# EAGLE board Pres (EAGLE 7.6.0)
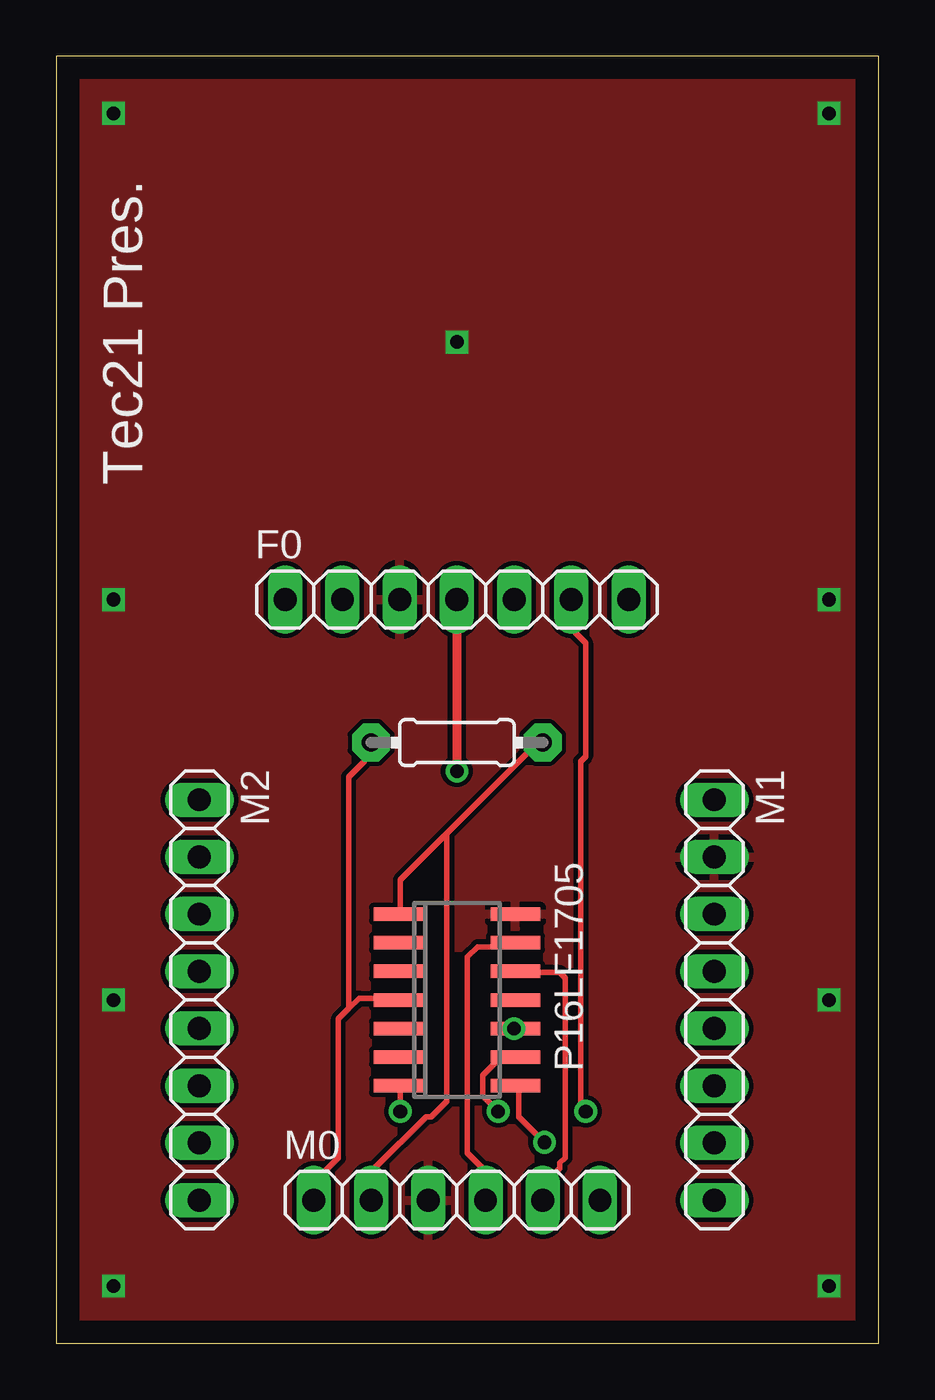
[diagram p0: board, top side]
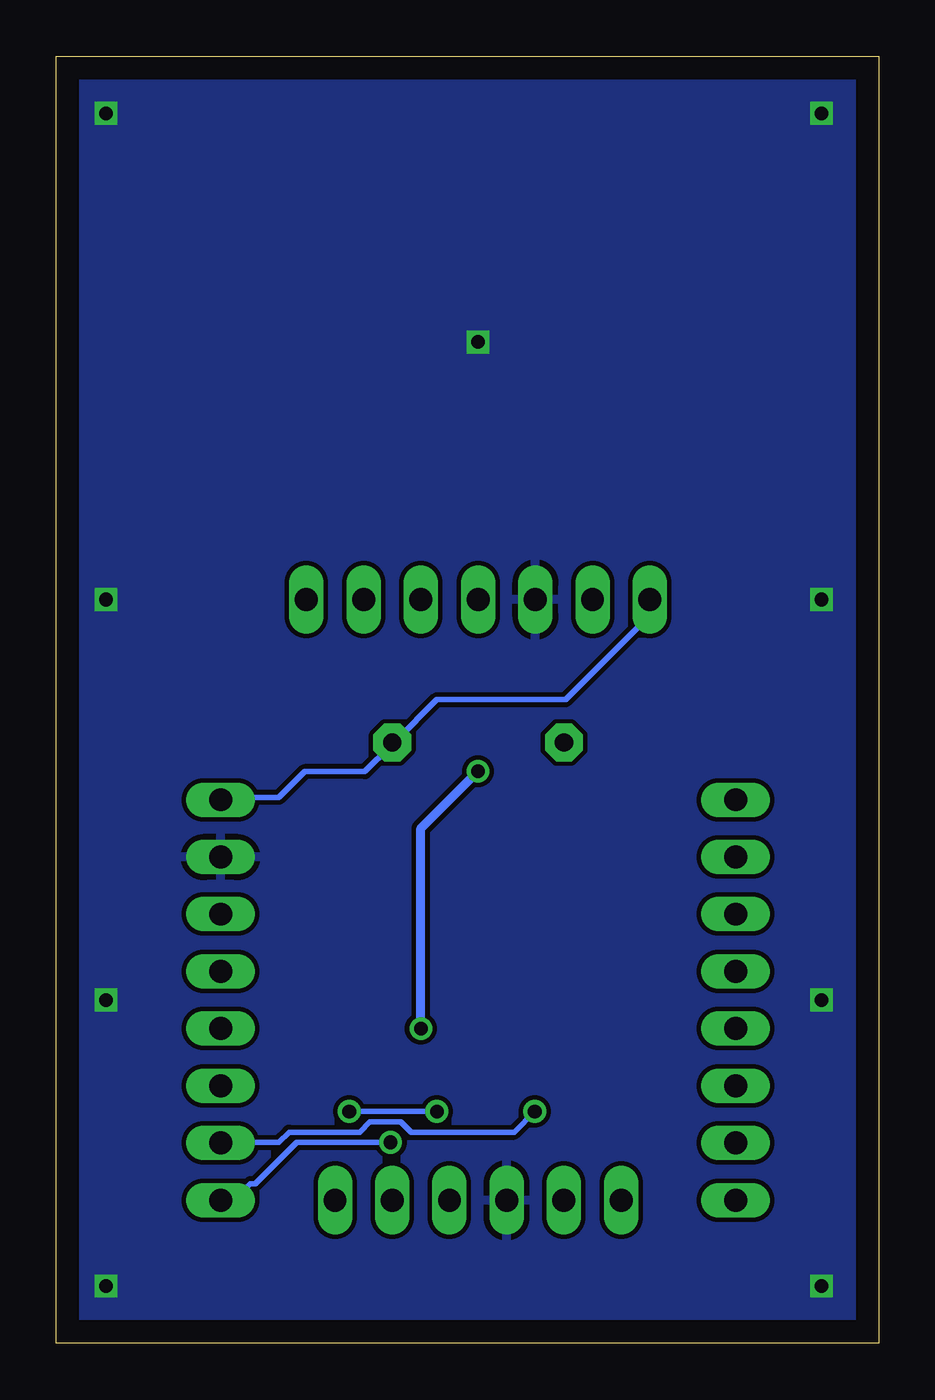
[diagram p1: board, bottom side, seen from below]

Size 36.5 x 57.14 mm. Coordinates in mm from the lower left corner, seen from the top.
Outline: 0,0 36.5,0 36.5,57.14 0,57.14 0,0
Copper layers (1*16): Top 0.035mm / dielectric 1.5mm / Bottom 0.035mm
Design rules "default": minimum track width 10mil, minimum drill 24mil, track to track 8mil, track to pad 8mil, pad to pad 8mil, via to via 8mil, smd to smd 8mil, copper to edge 40mil, drill to drill 8mil, minimum pad ring 10mil, minimum via ring 8mil, stop-mask expansion 4mil, vias tented up to drill 0mil, thermal gap 10mil

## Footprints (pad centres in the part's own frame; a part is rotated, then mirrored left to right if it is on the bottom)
0204/7 = drill 0.813 pad 1.676 octagon: 1 -3.81,0; 2 3.81,0
1X07 = drill 1.016 long: 1 -7.62,0; 2 -5.08,0; 3 -2.54,0; 4 0,0; 5 2.54,0; 6 5.08,0; 7 7.62,0
1X06 = drill 1.016 long: 1 -6.35,0; 2 -3.81,0; 3 -1.27,0; 4 1.27,0; 5 3.81,0; 6 6.35,0
1X08 = drill 1.016 long: 1 -8.89,0; 2 -6.35,0; 3 -3.81,0; 4 -1.27,0; 5 1.27,0; 6 3.81,0; 7 6.35,0; 8 8.89,0
SO-14 = smd 0.6 x 2.2: 1 -3.81,-2.6; 2 -2.54,-2.6; 3 -1.27,-2.6; 4 0,-2.6; 5 1.27,-2.6; 6 2.54,-2.6; 7 3.81,-2.6; 8 3.81,2.6; 9 2.54,2.6; 10 1.27,2.6; 11 0,2.6; 12 -1.27,2.6; 13 -2.54,2.6; 14 -3.81,2.6

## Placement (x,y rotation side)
10K  10k  [0204/7]  17.78,26.67 0 top
F0  [1X07]  17.78,33.02 0 top
M0  [1X06]  17.78,6.35 0 top
M1  [1X08]  29.21,15.24 270 top
M2  [1X08]  6.35,15.24 270 top
P16LF1705  PIC16F676SL  [SO-14]  17.78,15.24 270 top

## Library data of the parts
10K = adafruit
F0 M0 M1 M2 = pinhead
P16LF1705 = microchip; MF: MICROCHIP; MPN: PIC16F676-I/SL; OC_FARNELL: 9760520; OC_NEWARK: 92C4557

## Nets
CCL: M1.7 P16LF1705.7
CDA: M1.8 P16LF1705.8
GND: F0.3 M0.3 M1.2 P16LF1705.14
LCL: F0.6 P16LF1705.9
LDA: F0.4 P16LF1705.10
MCLR: 10K.1 M0.1 P16LF1705.4
N$8: F0.2
PGC: M0.5 P16LF1705.12
PGD: M0.4 P16LF1705.13
VDD: 10K.2 F0.1 M0.2 M1.1 P16LF1705.1

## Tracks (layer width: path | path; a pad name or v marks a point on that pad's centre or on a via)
CCL  (via drill 0.61)
  Top 0.254: v15.26,10.29 15.26,11.43 P16LF1705.7
  Bottom 0.254: v15.26,10.29 16.18,9.37 20.75,9.37 21.21,9.83 22.58,9.83 23.04,9.37 26.16,9.37 26.62,8.91 27.76,8.91 M1.7
CDA  (via drill 0.61)
  Top 0.254: v21.67,8.91 20.52,10.06 20.52,11.43 P16LF1705.8
  Bottom 0.254: v21.67,8.91 25.83,8.91 27.66,7.09 27.89,7.09 28.58,6.4 29.03,6.4 M1.8
GND  (via drill 0.6)
  other vias: 2.54,54.61 34.29,54.61 34.29,33.02 2.54,33.02 17.78,44.45 2.54,15.24 34.29,15.24 2.54,2.54 34.29,2.54
  pour Top: -1.27,58.42 38.1,58.42 38.1,-1.27 -1.27,-1.27
  pour Bottom: -1.27,58.42 38.1,58.42 38.1,-1.27 -1.27,-1.27
LCL  (via drill 0.61)
  Top 0.254: v19.61,10.29 18.92,10.97 18.92,11.89 19.61,12.57 20.3,12.57 P16LF1705.9 | v23.49,10.29 23.27,10.52 23.27,25.83 23.49,26.06 23.49,31.09 23.04,31.55 23.04,32.92 F0.6
  Bottom 0.254: v23.49,10.29 v19.61,10.29
LDA  (via drill 0.6)
  Top 0.254: P16LF1705.10 20.52,13.95 v20.32,13.97
  Top 0.406: F0.4 v17.78,25.4
  Bottom 0.406: v20.32,13.97 20.32,22.86 v17.78,25.4
MCLR
  Top 0.254: 12.98,14.86 12.52,14.4 12.52,8.23 11.61,7.32 11.61,6.4 M0.1 | 12.98,14.86 13.44,15.32 15.04,15.32 P16LF1705.4 | 12.98,14.86 12.98,25.15 13.67,25.83 13.67,26.29 13.89,26.52 10K.1
PGC
  Top 0.254: P16LF1705.12 20.52,16.46 22.35,16.46 22.58,16.23 22.58,8.23 22.35,8 22.35,7.77 21.67,7.09 21.67,6.4 M0.5
PGD
  Top 0.254: P16LF1705.13 20.3,17.6 18.69,17.6 18.24,17.14 18.24,8.46 19.15,7.54 19.15,6.4 M0.4
VDD
  Top 0.254: 17.32,22.63 21.44,26.75 10K.2 | 17.32,22.63 15.26,20.57 15.26,19.2 P16LF1705.1 | 17.32,22.63 17.32,10.74 16.64,10.06 16.41,10.06 14.12,7.77 14.12,6.4 M0.2
  Bottom 0.254: F0.1 10.24,32.92 10.69,32.46 10.69,31.77 13.89,28.57 19.61,28.57 21.44,26.75 10K.2 21.67,26.52 22.81,25.38 25.48,25.38 26.62,24.23 27.76,24.23 M1.1

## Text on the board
tPlace: Tec21 Pres.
